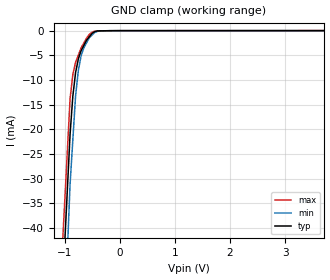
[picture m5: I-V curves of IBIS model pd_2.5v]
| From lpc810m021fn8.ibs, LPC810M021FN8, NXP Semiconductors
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[Model] pd_2.5v
Model_type Input
Vinl = 750.000mV
Vinh = 1.75000V
C_comp 587.000fF 585.000fF 589.000fF
| variable typ   min   max
[Voltage Range] 2.50000V 2.25000V 2.75000V
[POWER Clamp Reference] 2.50000V 2.25000V 2.75000V
[GND Clamp Reference] 0.00000V 0.00000V 0.00000V
[Temperature Range]   25   85   -40
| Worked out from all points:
|   GND clamp passes 1 mA (typ) near -0.53 V on its own axis
[GND Clamp]
-2.5V     -385.6mA   -472.2mA   -357.5mA
-900mV    -20.98mA   -31.13mA   -13.8mA
-850mV    -13.28mA   -22.15mA   -8.911mA
-800mV    -8.483mA   -13.16mA   -6.412mA
-750mV    -5.729mA   -8.059mA   -4.946mA
-700mV    -4.056mA   -5.078mA   -3.479mA
-650mV    -2.988mA   -3.465mA   -2.487mA
-550mV    -1.226mA   -1.411mA   -758.6uA
-500mV    -532.9uA   -883.1uA   -295.9uA
-400mV    -46.91uA   -121.5uA   -71.69uA
-200mV    -8.97uA    -6.932uA   -21.03uA
5V        8.051uA    7.985uA    18.06uA
[POWER Clamp]
-2.5V     0A         0A         0A
5V        0A         0A         0A
